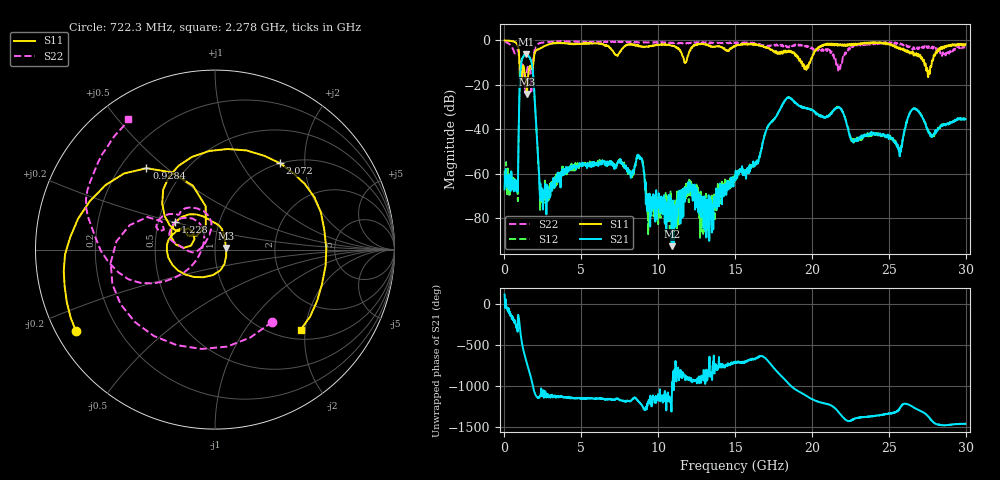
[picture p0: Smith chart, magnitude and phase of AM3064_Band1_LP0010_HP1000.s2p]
# Hz S DB R 50.0
!freq dBS11 angS11 dBS21 angS21 dBS12 angS12 dBS22 angS22
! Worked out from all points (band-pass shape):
!   1600 points, 10 MHz to 29.98 GHz, reference 50 ohm
!   highest |S21| = -6.21 dB at 1.397 GHz (marker M1); lowest = -92.5 dB at 10.88 GHz (marker M2)
!   |S21| within 3 dB of the highest: 1.117 GHz to 1.732 GHz (615.4 MHz wide, 43.2 % of centre)
!   lowest |S11| = -24.1 dB at 1.453 GHz (marker M3), VSWR 1.13, Z = 56.6 + j0.963 ohm
!   |S11| at or under -10 dB: 973.7 MHz to 1.877 GHz (903.4 MHz wide, 63.4 % of centre); 19.35 GHz to 19.82 GHz (467.6 MHz wide, 2.39 % of centre); 27.3 GHz to 27.79 GHz (495.7 MHz wide, 1.8 % of centre)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
!   |S22| runs from -23.6 to -0.3 dB; largest |S21 - S12| = 0.0059
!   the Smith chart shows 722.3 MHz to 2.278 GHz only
!   S11 on the Smith chart (normalised r, x): 722.3 MHz: 0.06, -0.27; 928.4 MHz: 0.31, +0.43; 1.228 GHz: 0.61, +0.20; 2.072 GHz: 0.99, +1.50; 2.278 GHz: 1.21, -1.89
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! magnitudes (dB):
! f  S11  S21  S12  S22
! 10 MHz  0.0  -67.0  -58.6  -0.3
! 722.3 MHz  -0.9  -62.8  -61.9  -5.8
! 928.4 MHz  -4.5  -39.6  -39.8  -6.1
! 1.228 GHz  -11.4  -7.3  -7.3  -12.0
! 1.397 GHz  -18.2  -6.2  -6.2  -18.0
! 1.453 GHz  -24.1  -6.3  -6.3  -14.6
! 1.791 GHz  -13.1  -10.9  -10.9  -17.6
! 2.072 GHz  -4.4  -39.2  -39.2  -2.3
! 2.278 GHz  -3.7  -66.3  -65.7  -1.2
! 5.015 GHz  -1.4  -55.8  -55.8  -0.8
! 8.801 GHz  -2.7  -52.2  -52.8  -0.9
! 9.344 GHz  -2.7  -76.0  -87.1  -0.9
! 10 GHz  -2.0  -74.0  -82.6  -0.9
! 10.88 GHz  -2.5  -92.5  -76.3  -1.1
! 15 GHz  -2.7  -63.1  -60.4  -1.3
! 18.34 GHz  -5.5  -26.1  -26.1  -2.7
! 19.99 GHz  -8.2  -31.3  -31.4  -3.4
! 25 GHz  -1.4  -44.4  -42.9  -1.1
! 25.75 GHz  -3.6  -49.9  -49.8  -1.7
! 26.64 GHz  -6.5  -30.8  -30.6  -3.6
! 27.56 GHz  -16.5  -40.7  -40.4  -2.8
! 29.98 GHz  -1.7  -35.4  -35.0  -3.2
